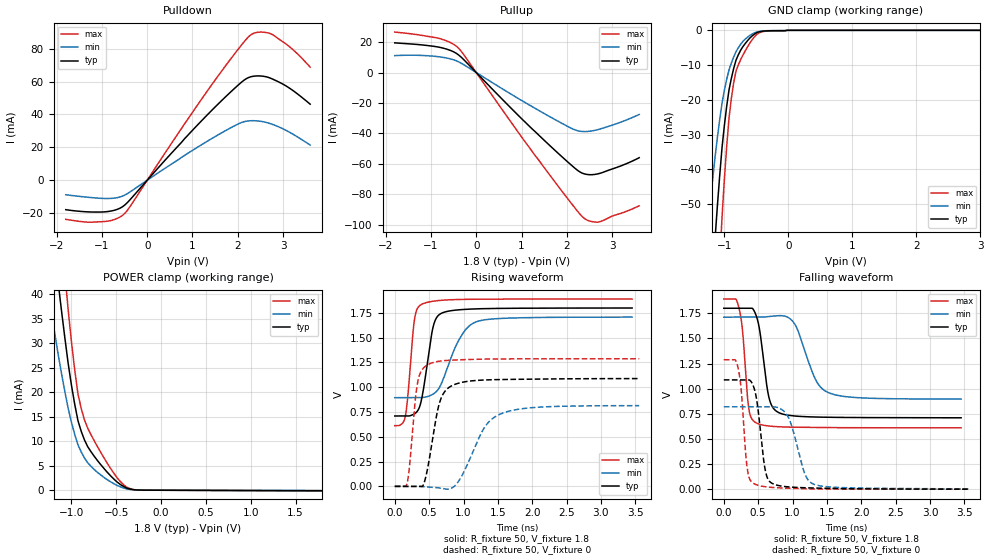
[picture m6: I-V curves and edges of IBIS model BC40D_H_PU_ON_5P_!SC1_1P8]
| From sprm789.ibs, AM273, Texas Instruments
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|   Model Cell BC40D_H_PU_ON_5P_!SC1_1P8
|BC40D_H_PU_ON_5P_!SC1_1P8
[Model]   BC40D_H_PU_ON_5P_!SC1_1P8
Model_type   I/O
Polarity   Non-Inverting
Enable   Active-Low
Vinl =  0.63
Vinh =  1.17
Cref =  15pF
Rref =  100.0000M
Vref =  0V
Vmeas =  0.9
C_comp   2.364487p   2.290698p   2.389419p
|[Input load] weak_pu_on
|[Output drive] fast
|[supplytol] 5
|[temp] ind
[Model Spec]
Vinl   0.63   0.5985   0.6615
Vinh   1.17   1.1115   1.2285
[Temperature Range]   25   125   -40
[Voltage Range]   1.8   1.71   1.89
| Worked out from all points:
|   slope of the pulldown table from 0 to 0.27 V, typ, clamps not added: 32.2 ohm
|   slope of the pullup table from 0 to 0.27 V, typ, clamps not added: 32.5 ohm
|   GND clamp passes 1 mA (typ) near -0.52 V on its own axis
|   POWER clamp passes 1 mA (typ) near -0.44 V on its own axis
|   rising waveform, R_fixture 50, V_fixture 1.8: 20-80 % time 145ps typ, 302ps min, 93.4ps max; typ from 0.71 V to 1.8 V
|   rising waveform, R_fixture 50, V_fixture 0: 20-80 % time 176ps typ, 353ps min, 106ps max; typ from 0 V to 1.09 V
|   falling waveform, R_fixture 50, V_fixture 1.8: 20-80 % time 130ps typ, 266ps min, 88.1ps max; typ from 1.8 V to 0.711 V
|   falling waveform, R_fixture 50, V_fixture 0: 20-80 % time 113ps typ, 198ps min, 84.3ps max; typ from 1.09 V to 0.002 V
| Nom Voltages:
|   VDD=1.1, VDDS=1.8, VDDS18=1.8, ESD_BIASFET=0, VSS=0, VSSS=0
| Min Voltages:
|   VDD=1.045, VDDS=1.71, VDDS18=1.71, ESD_BIASFET=0, VSS=0, VSSS=0
| Max Voltages:
|   VDD=1.16, VDDS=1.89, VDDS18=1.89, ESD_BIASFET=0, VSS=0, VSSS=0
[POWER_clamp]
|   voltage   I(typ)   I(min)   I(max)
-1.8V     158.8mA    112.5mA    219.8mA
-1.255V   59.97mA    40.01mA    84.91mA
-1.145V   41.92mA    27.41mA    59.76mA
-1.109V   36.32mA    23.62mA    51.83mA
-1.073V   30.96mA    20.04mA    44.16mA
-1.036V   25.83mA    16.67mA    36.76mA
-963.6mV  17.54mA    11.39mA    24.56mA
-890.9mV  12.01mA    7.798mA    16.67mA
-818.2mV  8.875mA    5.598mA    12.64mA
-563.6mV  2.954mA    1.726mA    4.46mA
-272.7mV  55.97uA    39.54uA    57.56uA
1.8V      -99.94uA   -59.14uA   -145.1uA
[Pulldown]
|   voltage   I(typ)   I(min)   I(max)
-1.8V     -17.92mA   -8.85mA    -23.8mA
-1.309V   -19.26mA   -10.37mA   -25.51mA
-927.3mV  -19.22mA   -11.12mA   -25.08mA
-654.5mV  -17.65mA   -10.56mA   -23.13mA
-490.9mV  -14.97mA   -8.985mA   -20.05mA
1.364V    40.78mA    24.32mA    55.7mA
2.073V    59.41mA    35mA       81.9mA
2.291V    62.96mA    36.2mA     88.48mA
2.509V    63.41mA    35.84mA    90.12mA
2.782V    61.38mA    33.82mA    88.42mA
3.218V    54.59mA    28.02mA    79.45mA
3.6V      46.26mA    21.39mA    68.79mA
[Pullup]
|   voltage   I(typ)   I(min)   I(max)
-1.8V     19.47mA    11.11mA    26.55mA
-818.2mV  16.61mA    10.32mA    22.37mA
-545.5mV  14.21mA    8.765mA    19.31mA
-381.8mV  11.35mA    6.928mA    15.71mA
1.255V    -37.58mA   -22.7mA    -52.59mA
2.127V    -61.49mA   -36.97mA   -86.91mA
2.291V    -65.3mA    -38.55mA   -92.97mA
2.4V      -66.65mA   -38.77mA   -96.07mA
2.564V    -67.08mA   -38.3mA    -97.93mA
2.727V    -66.24mA   -37.15mA   -97.99mA
3.273V    -60.4mA    -31.68mA   -91.65mA
3.6V      -55.92mA   -27.55mA   -87.52mA
[GND_clamp]
|   voltage   I(typ)   I(min)   I(max)
-1.8V     -270.2mA   -170.2mA   -430.1mA
-1.255V   -91.68mA   -55.92mA   -148.5mA
-1.145V   -59.94mA   -36.46mA   -97.14mA
-1.109V   -50.51mA   -30.84mA   -81.61mA
-1.073V   -41.77mA   -25.67mA   -67.13mA
-1.036V   -33.71mA   -20.95mA   -53.68mA
-927.3mV  -17.15mA   -11.38mA   -25.19mA
-854.5mV  -10.96mA   -7.663mA   -15.08mA
-781.8mV  -7.031mA   -5.001mA   -9.947mA
-563.6mV  -1.569mA   -1.041mA   -2.641mA
-18.18mV  0A         0A         0A
3.6V      0A         0A         0A
[Ramp]
| variable   typ   min   max
dV/dt_f 0.66463159/0.13264729n  0.4990718/0.27161645n  0.7761677/89.737884p
dV/dt_r 0.66384732/0.17820849n  0.5092724/0.36663744n 0.78038296/0.10684153n
R_load = 50
[Rising Waveform]
R_fixture = 50
V_fixture = 1.8
V_fixture_min = 1.71
V_fixture_max = 1.89
|   time   V(typ)   V(min)   V(max)
0s        710.5mV    895.2mV    613.1mV
151.7ps   710.5mV    895.2mV    701.4mV
187ps     710.5mV    895.2mV    890mV
286.2ps   732.2mV    895.2mV    1.681V
390.1ps   878.6mV    896.9mV    1.837V
553.7ps   1.597V     929.4mV    1.868V
686.5ps   1.749V     1.05V      1.878V
948.8ps   1.783V     1.497V     1.886V
1.197ns   1.791V     1.663V     1.888V
3.453ns   1.8V       1.708V     1.89V
[Rising Waveform]
R_fixture = 50
V_fixture = 0
V_fixture_min = 0
V_fixture_max = 0
|   time   V(typ)   V(min)   V(max)
0s        0V         0V         2.427mV
178.8ps   0V         0V         31.25mV
328.8ps   0V         0V         1.035V
405.2ps   0V         -2.984mV   1.184V
485.8ps   210mV      -7.093mV   1.23V
655.6ps   853.6mV    -16.4mV    1.264V
861ps     1.026V     -2.093mV   1.275V
1.312ns   1.074V     601.9mV    1.284V
1.533ns   1.078V     729mV      1.286V
3.556ns   1.088V     814.8mV    1.288V
[Falling Waveform]
R_fixture = 50
V_fixture = 1.8
V_fixture_min = 1.71
V_fixture_max = 1.89
|   time   V(typ)   V(min)   V(max)
0s        1.799V     1.711V     1.891V
218.1ps   1.799V     1.711V     1.81V
270.7ps   1.799V     1.711V     1.592V
362.3ps   1.799V     1.711V     810.1mV
472.5ps   1.724V     1.711V     660.7mV
652.6ps   926mV      1.717V     629.8mV
801.1ps   762.2mV    1.726V     622.1mV
1.032ns   729.1mV    1.643V     617.8mV
1.52ns    716.5mV    962.1mV    613.8mV
3.453ns   711.4mV    897.1mV    611.7mV
[Falling Waveform]
R_fixture = 50
V_fixture = 0
V_fixture_min = 0
V_fixture_max = 0
|   time   V(typ)   V(min)   V(max)
0s        1.088V     820.4mV    1.288V
203.8ps   1.088V     820.4mV    1.217V
254.1ps   1.088V     820.4mV    984.5mV
341.4ps   1.088V     820.4mV    207mV
444.1ps   998.5mV    820.4mV    55.38mV
602.1ps   195.2mV    820.4mV    26.75mV
715.3ps   55.69mV    820.4mV    19.07mV
935.6ps   25.31mV    720.9mV    11.95mV
1.302ns   13.89mV    53.39mV    5.238mV
3.556ns   2.477mV    5.118mV    2.437mV
